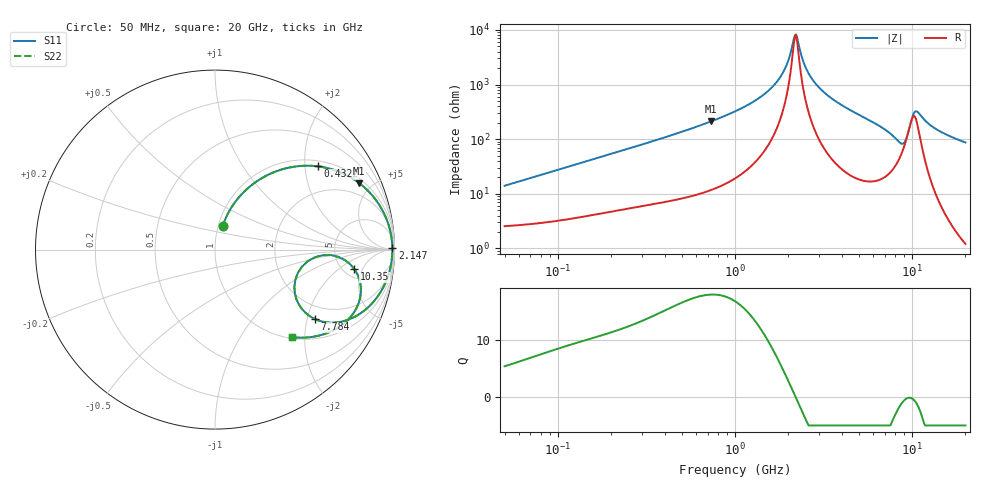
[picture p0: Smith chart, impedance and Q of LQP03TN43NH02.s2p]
!Murata Part Number: LQP03TN43NH02
!These Parameters are Measured in Series Mode Connection
!  o--[Z]--o
!Port1  Port2
!  o-------o
!Freq. Start=50[MHz] Stop=20[GHz], 401[Steps]
# Hz S RI R 50
!Freq.(Hz) S11(Real) S11(Imag) S21(Real) S21(Imag) S12(Real) S12(Imag) S22(Real) S22(Imag)
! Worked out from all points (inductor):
!   401 points, 50 MHz to 20 GHz, reference 50 ohm
!   read as one part in series: L = 43.8 nH near 51.52 MHz
!   highest Q = 18 at 730.1 MHz (marker M1), where L = 45.8 nH
!   self-resonance near 2.179 GHz
!   S11 on the Smith chart (normalised r, x): 50 MHz: 1.05, +0.28; 432.2 MHz: 1.15, +2.33; 2.147 GHz: open; 7.784 GHz: 1.56, -2.24; 10.35 GHz: 6.24, -3.53; 20 GHz: 1.02, -1.74
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5e7  0.0423 0.1291  0.9577 -0.1291  0.9577 -0.1291  0.0423 0.1291
1.364002e8  0.1449 0.3046  0.8551 -0.3046  0.8551 -0.3046  0.1449 0.3046
3.721004e8  0.4993 0.4672  0.5007 -0.4672  0.5007 -0.4672  0.4993 0.4672
4.322267e8  0.572 0.4639  0.428 -0.4639  0.428 -0.4639  0.572 0.4639
7.30116e8  0.8031 0.3709  0.1969 -0.3709  0.1969 -0.3709  0.8031 0.3709
1e9  0.8987 0.2735  0.1013 -0.2735  0.1013 -0.2735  0.8987 0.2735
1.369645e9  0.9574 0.1655  0.0426 -0.1655  0.0426 -0.1655  0.9574 0.1655
1.689197e9  0.9787 0.0924  0.0213 -0.0924  0.0213 -0.0924  0.9787 0.0924
1.932977e9  0.9859 0.0453  0.0141 -0.0453  0.0141 -0.0453  0.9859 0.0453
2.146657e9  0.9881 0.00858  0.0119 -0.00858  0.0119 -0.00858  0.9881 0.00858
2.245319e9  0.9881 -0.00722  0.0119 0.00722  0.0119 0.00722  0.9881 -0.00722
2.456456e9  0.9866 -0.039  0.0134 0.039  0.0134 0.039  0.9866 -0.039
2.728004e9  0.9819 -0.0764  0.0181 0.0764  0.0181 0.0764  0.9819 -0.0764
3.850025e9  0.941 -0.2034  0.059 0.2034  0.059 0.2034  0.941 -0.2034
5.683258e9  0.8175 -0.3505  0.1825 0.3505  0.1825 0.3505  0.8175 -0.3505
7.442007e9  0.6121 -0.4039  0.3879 0.4039  0.3879 0.4039  0.6121 -0.4039
7.784049e9  0.5582 -0.3875  0.4418 0.3875  0.4418 0.3875  0.5582 -0.3875
8.907419e9  0.4473 -0.1694  0.5527 0.1694  0.5527 0.1694  0.4473 -0.1694
9.600142e9  0.6019 -0.0309  0.3981 0.0309  0.3981 0.0309  0.6019 -0.0309
1.034674e10  0.7769 -0.1089  0.2231 0.1089  0.2231 0.1089  0.7769 -0.1089
1.334722e10  0.7067 -0.4207  0.2933 0.4207  0.2933 0.4207  0.7067 -0.4207
2e10  0.4315 -0.4884  0.5685 0.4884  0.5685 0.4884  0.4315 -0.4884
